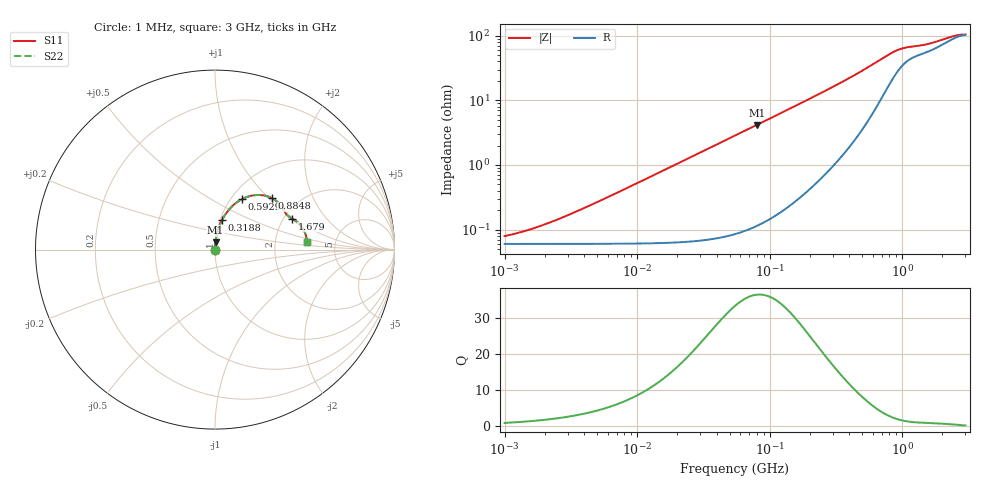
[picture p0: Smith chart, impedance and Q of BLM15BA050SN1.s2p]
! BLM15BA050SN1
# Hz S RI R 50
!Freq.(Hz) S11(Real) S11(Imag) S21(Real) S21(Imag) S12(Real) S12(Imag) S22(Real) S22(Imag)
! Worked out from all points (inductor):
!   401 points, 1 MHz to 3 GHz, reference 50 ohm
!   read as one part in series: L = 8.27 nH near 3.529 MHz
!   highest Q = 36.6 at 80.12 MHz (marker M1), where L = 8.29 nH
!   S11 on the Smith chart (normalised r, x): 1 MHz: 1.00, +0.00; 318.8 MHz: 1.02, +0.34; 592.9 MHz: 1.12, +0.70; 884.8 MHz: 1.49, +1.05; 1.679 GHz: 2.21, +0.97; 3 GHz: 3.07, +0.34
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1000000  0.0006 0.000519  0.9994 -0.000519  0.9994 -0.000519  0.0006 0.000519
1323425  0.0006 0.000687  0.9994 -0.000687  0.9994 -0.000687  0.0006 0.000687
1822989  0.000601 0.000946  0.9994 -0.000946  0.9994 -0.000946  0.000601 0.000946
2561897  0.000602 0.00133  0.9994 -0.00133  0.9994 -0.00133  0.000602 0.00133
3823119  0.000605 0.00198  0.9994 -0.00198  0.9994 -0.00198  0.000605 0.00198
1.461624e7  0.000675 0.00758  0.9993 -0.00758  0.9993 -0.00758  0.000675 0.00758
5.477226e7  0.00166 0.0284  0.9983 -0.0284  0.9983 -0.0284  0.00166 0.0284
8.011685e7  0.00287 0.0416  0.9971 -0.0416  0.9971 -0.0416  0.00287 0.0416
1.348146e8  0.00708 0.0699  0.9929 -0.0699  0.9929 -0.0699  0.00708 0.0699
2.094008e8  0.0165 0.1084  0.9835 -0.1084  0.9835 -0.1084  0.0165 0.1084
3.188066e8  0.0388 0.1639  0.9612 -0.1639  0.9612 -0.1639  0.0388 0.1639
4.480278e8  0.0806 0.2258  0.9194 -0.2258  0.9194 -0.2258  0.0806 0.2258
5.929311e8  0.1503 0.2812  0.8497 -0.2812  0.8497 -0.2812  0.1503 0.2812
6.958997e8  0.2119 0.302  0.7881 -0.302  0.7881 -0.302  0.2119 0.302
8.005644e8  0.2752 0.3012  0.7248 -0.3012  0.7248 -0.3012  0.2752 0.3012
8.848309e8  0.318 0.2862  0.682 -0.2862  0.682 -0.2862  0.318 0.2862
1.080907e9  0.3738 0.2357  0.6262 -0.2357  0.6262 -0.2357  0.3738 0.2357
1.294266e9  0.395 0.2003  0.605 -0.2003  0.605 -0.2003  0.395 0.2003
1.67892e9  0.4288 0.1731  0.5712 -0.1731  0.5712 -0.1731  0.4288 0.1731
2.177892e9  0.4777 0.1329  0.5223 -0.1329  0.5223 -0.1329  0.4777 0.1329
2.607784e9  0.5044 0.0857  0.4956 -0.0857  0.4956 -0.0857  0.5044 0.0857
3e9  0.5115 0.0408  0.4885 -0.0408  0.4885 -0.0408  0.5115 0.0408
